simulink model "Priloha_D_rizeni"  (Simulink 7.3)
settings: Solver=ode45  StartTime=0.0  StopTime=0.7  FixedStep=0.6e-3  MaxStep=0.08e-3  RelTol=0.8e-3
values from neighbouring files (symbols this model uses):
  ILi = [0 Imax]    [Priloha_B_motor1_parametry.m]    (also in Priloha_C_motor2_parametry.m)
  Im = Psim / Ldi(1)    [Priloha_B_motor1_parametry.m]    (also in Priloha_C_motor2_parametry.m)
  Imax = 8    [Priloha_B_motor1_parametry.m]    (also in Priloha_C_motor2_parametry.m)
  J = 7e-3    (= 0.007)    [Priloha_B_motor1_parametry.m]    (also in Priloha_C_motor2_parametry.m)
  Kiid = 1 / (KM * 2 * tausigmaid / Rs)    (= 1975)    [Priloha_B_motor1_parametry.m]    (also in Priloha_C_motor2_parametry.m)
  Kiiq = 1 / (KM * 2 * tausigmaiq / Rs)    (= 1975)    [Priloha_B_motor1_parametry.m]    (also in Priloha_C_motor2_parametry.m)
  Kiwq = 1 / (Psim * p * 8 * (2 * tausigmaiq)^2 / J)    (= 306.115309264)    [Priloha_B_motor1_parametry.m]    (also in Priloha_C_motor2_parametry.m = 402.854511971)
  KM = 1    [Priloha_B_motor1_parametry.m]    (also in Priloha_C_motor2_parametry.m)
  Kpid = Ldi(1) / (KM * 2 * tausigmaid)    [Priloha_B_motor1_parametry.m]    (also in Priloha_C_motor2_parametry.m)
  Kpiq = Lqi(1) / (KM * 2 * tausigmaiq)    [Priloha_B_motor1_parametry.m]    (also in Priloha_C_motor2_parametry.m)
  Kpwq = 4 / (Psim * p * 8 * (2 * tausigmaiq) / J)    (= 2.44892247411)    [Priloha_B_motor1_parametry.m]    (also in Priloha_C_motor2_parametry.m = 3.22283609576)
  Ld = 22.5e-3    (= 0.0225)    [Priloha_B_motor1_parametry.m]    (also in Priloha_C_motor2_parametry.m)
  Ldi = [Ldi Ldi]    [Priloha_B_motor1_parametry.m]    (also in Priloha_C_motor2_parametry.m)
  Lq = 54e-3    (= 0.054)    [Priloha_B_motor1_parametry.m]    (also in Priloha_C_motor2_parametry.m)
  Lqi = [Lqi Lqi]    [Priloha_B_motor1_parametry.m]    (also in Priloha_C_motor2_parametry.m)
  p = 3    [Priloha_B_motor1_parametry.m]    (also in Priloha_C_motor2_parametry.m)
  Psim = 238.2e-3    (= 0.2382)    [Priloha_B_motor1_parametry.m]    (also in Priloha_C_motor2_parametry.m = 0.181)
  Rs = 3.95    [Priloha_B_motor1_parametry.m]    (also in Priloha_C_motor2_parametry.m)
  tausigmaid = 1 / fM    (= 0.001)    [Priloha_B_motor1_parametry.m]    (also in Priloha_C_motor2_parametry.m)
  tausigmaiq = 1 / fM    (= 0.001)    [Priloha_B_motor1_parametry.m]    (also in Priloha_C_motor2_parametry.m)
  Umax = 115    [Priloha_B_motor1_parametry.m]    (also in Priloha_C_motor2_parametry.m)
undefined symbols (not defined in the file or in its folder): Floor, magnitude
libraries: simulink x21
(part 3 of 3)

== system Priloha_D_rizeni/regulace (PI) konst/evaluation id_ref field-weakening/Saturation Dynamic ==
  up : Inport  OutDataType=fixdt(1, 16)  OutScaling=2^0
  u : Inport  Port=2  OutDataType=fixdt(1, 16)  OutScaling=2^0
  lo : Inport  Port=3  OutDataType=fixdt(1, 16)  OutScaling=2^0
  Data Type Duplicate : simulink/Signal Attributes/Data Type Duplicate  NumInputPorts=2
  Data Type Propagation : simulink/Signal Attributes/Data Type Propagation  PropDataType=fixdt(1, 16)  IfRefDouble=double  IfRefSingle=single  IsSigned=IsSigned1  NumBitsBase=NumBits1  NumBitsMult=1  NumBitsAdd=0  NumBitsAllowFinal=1:128  PropScaling=2^-10  ValuesUsedBestPrec=[5 -7]  SlopeBase=Slope1  SlopeMult=1  SlopeAdd=0  BiasBase=Bias1  BiasMult=1  BiasAdd=0
  LowerRelop1 : RelationalOperator  DisableCoverage=on  Operator=>  LogicOutDataTypeMode=boolean  LogicDataType=fixdt(0, 8)  OutDataTypeStr=boolean
  Switch : Switch  Criteria=u2 ~= 0  OutDataType=fixdt(1, 16)  OutScaling=2^0  OutDataTypeStr=Inherit: Inherit via back propagation  ZeroCross=off
  Switch2 : Switch  Criteria=u2 ~= 0  OutMin=OutMin  OutMax=OutMax  OutDataType=OutDataType  OutScaling=OutScaling  OutDataTypeStr=Inherit: Inherit via back propagation  ZeroCross=off
  UpperRelop : RelationalOperator  DisableCoverage=on  Operator=<  LogicOutDataTypeMode=boolean  LogicDataType=fixdt(0, 8)  OutDataTypeStr=boolean
  y1 : Outport  OutMin=OutMin  OutMax=OutMax  OutDataType=fixdt(1, 16)  OutScaling=2^0
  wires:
  up/1 -> Switch2/1, LowerRelop1/2
  u/1 -> Data Type Propagation/2, Data Type Propagation/1, LowerRelop1/1, Switch/3, UpperRelop/1
  lo/1 -> Switch/1, UpperRelop/2
  Switch/1 -> Data Type Duplicate/2, Switch2/3, Data Type Propagation/3
  Switch2/1 -> Data Type Duplicate/1, y1/1
  LowerRelop1/1 -> Switch2/2
  UpperRelop/1 -> Switch/2

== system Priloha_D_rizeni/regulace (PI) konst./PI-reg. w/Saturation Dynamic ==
  up : Inport  OutDataType=fixdt(1, 16)  OutScaling=2^0
  u : Inport  Port=2  OutDataType=fixdt(1, 16)  OutScaling=2^0
  lo : Inport  Port=3  OutDataType=fixdt(1, 16)  OutScaling=2^0
  Data Type Duplicate : simulink/Signal Attributes/Data Type Duplicate  NumInputPorts=2
  Data Type Propagation : simulink/Signal Attributes/Data Type Propagation  PropDataType=fixdt(1, 16)  IfRefDouble=double  IfRefSingle=single  IsSigned=IsSigned1  NumBitsBase=NumBits1  NumBitsMult=1  NumBitsAdd=0  NumBitsAllowFinal=1:128  PropScaling=2^-10  ValuesUsedBestPrec=[5 -7]  SlopeBase=Slope1  SlopeMult=1  SlopeAdd=0  BiasBase=Bias1  BiasMult=1  BiasAdd=0
  LowerRelop1 : RelationalOperator  DisableCoverage=on  Operator=>  LogicOutDataTypeMode=boolean  LogicDataType=fixdt(0, 8)  OutDataTypeStr=boolean
  Switch : Switch  Criteria=u2 ~= 0  OutDataType=fixdt(1, 16)  OutScaling=2^0  OutDataTypeStr=Inherit: Inherit via back propagation  ZeroCross=off
  Switch2 : Switch  Criteria=u2 ~= 0  OutMin=OutMin  OutMax=OutMax  OutDataType=OutDataType  OutScaling=OutScaling  OutDataTypeStr=Inherit: Inherit via back propagation  ZeroCross=off
  UpperRelop : RelationalOperator  DisableCoverage=on  Operator=<  LogicOutDataTypeMode=boolean  LogicDataType=fixdt(0, 8)  OutDataTypeStr=boolean
  y1 : Outport  OutMin=OutMin  OutMax=OutMax  OutDataType=fixdt(1, 16)  OutScaling=2^0
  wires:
  up/1 -> Switch2/1, LowerRelop1/2
  u/1 -> Data Type Propagation/2, Data Type Propagation/1, LowerRelop1/1, Switch/3, UpperRelop/1
  lo/1 -> Switch/1, UpperRelop/2
  Switch/1 -> Data Type Duplicate/2, Switch2/3, Data Type Propagation/3
  Switch2/1 -> Data Type Duplicate/1, y1/1
  LowerRelop1/1 -> Switch2/2
  UpperRelop/1 -> Switch/2

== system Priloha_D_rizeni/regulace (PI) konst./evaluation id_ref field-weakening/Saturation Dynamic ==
  up : Inport  OutDataType=fixdt(1, 16)  OutScaling=2^0
  u : Inport  Port=2  OutDataType=fixdt(1, 16)  OutScaling=2^0
  lo : Inport  Port=3  OutDataType=fixdt(1, 16)  OutScaling=2^0
  Data Type Duplicate : simulink/Signal Attributes/Data Type Duplicate  NumInputPorts=2
  Data Type Propagation : simulink/Signal Attributes/Data Type Propagation  PropDataType=fixdt(1, 16)  IfRefDouble=double  IfRefSingle=single  IsSigned=IsSigned1  NumBitsBase=NumBits1  NumBitsMult=1  NumBitsAdd=0  NumBitsAllowFinal=1:128  PropScaling=2^-10  ValuesUsedBestPrec=[5 -7]  SlopeBase=Slope1  SlopeMult=1  SlopeAdd=0  BiasBase=Bias1  BiasMult=1  BiasAdd=0
  LowerRelop1 : RelationalOperator  DisableCoverage=on  Operator=>  LogicOutDataTypeMode=boolean  LogicDataType=fixdt(0, 8)  OutDataTypeStr=boolean
  Switch : Switch  Criteria=u2 ~= 0  OutDataType=fixdt(1, 16)  OutScaling=2^0  OutDataTypeStr=Inherit: Inherit via back propagation  ZeroCross=off
  Switch2 : Switch  Criteria=u2 ~= 0  OutMin=OutMin  OutMax=OutMax  OutDataType=OutDataType  OutScaling=OutScaling  OutDataTypeStr=Inherit: Inherit via back propagation  ZeroCross=off
  UpperRelop : RelationalOperator  DisableCoverage=on  Operator=<  LogicOutDataTypeMode=boolean  LogicDataType=fixdt(0, 8)  OutDataTypeStr=boolean
  y1 : Outport  OutMin=OutMin  OutMax=OutMax  OutDataType=fixdt(1, 16)  OutScaling=2^0
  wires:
  up/1 -> Switch2/1, LowerRelop1/2
  u/1 -> Data Type Propagation/2, Data Type Propagation/1, LowerRelop1/1, Switch/3, UpperRelop/1
  lo/1 -> Switch/1, UpperRelop/2
  Switch/1 -> Data Type Duplicate/2, Switch2/3, Data Type Propagation/3
  Switch2/1 -> Data Type Duplicate/1, y1/1
  LowerRelop1/1 -> Switch2/2
  UpperRelop/1 -> Switch/2

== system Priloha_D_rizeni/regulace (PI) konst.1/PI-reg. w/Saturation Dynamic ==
  up : Inport  OutDataType=fixdt(1, 16)  OutScaling=2^0
  u : Inport  Port=2  OutDataType=fixdt(1, 16)  OutScaling=2^0
  lo : Inport  Port=3  OutDataType=fixdt(1, 16)  OutScaling=2^0
  Data Type Duplicate : simulink/Signal Attributes/Data Type Duplicate  NumInputPorts=2
  Data Type Propagation : simulink/Signal Attributes/Data Type Propagation  PropDataType=fixdt(1, 16)  IfRefDouble=double  IfRefSingle=single  IsSigned=IsSigned1  NumBitsBase=NumBits1  NumBitsMult=1  NumBitsAdd=0  NumBitsAllowFinal=1:128  PropScaling=2^-10  ValuesUsedBestPrec=[5 -7]  SlopeBase=Slope1  SlopeMult=1  SlopeAdd=0  BiasBase=Bias1  BiasMult=1  BiasAdd=0
  LowerRelop1 : RelationalOperator  DisableCoverage=on  Operator=>  LogicOutDataTypeMode=boolean  LogicDataType=fixdt(0, 8)  OutDataTypeStr=boolean
  Switch : Switch  Criteria=u2 ~= 0  OutDataType=fixdt(1, 16)  OutScaling=2^0  OutDataTypeStr=Inherit: Inherit via back propagation  ZeroCross=off
  Switch2 : Switch  Criteria=u2 ~= 0  OutMin=OutMin  OutMax=OutMax  OutDataType=OutDataType  OutScaling=OutScaling  OutDataTypeStr=Inherit: Inherit via back propagation  ZeroCross=off
  UpperRelop : RelationalOperator  DisableCoverage=on  Operator=<  LogicOutDataTypeMode=boolean  LogicDataType=fixdt(0, 8)  OutDataTypeStr=boolean
  y1 : Outport  OutMin=OutMin  OutMax=OutMax  OutDataType=fixdt(1, 16)  OutScaling=2^0
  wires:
  up/1 -> Switch2/1, LowerRelop1/2
  u/1 -> Data Type Propagation/2, Data Type Propagation/1, LowerRelop1/1, Switch/3, UpperRelop/1
  lo/1 -> Switch/1, UpperRelop/2
  Switch/1 -> Data Type Duplicate/2, Switch2/3, Data Type Propagation/3
  Switch2/1 -> Data Type Duplicate/1, y1/1
  LowerRelop1/1 -> Switch2/2
  UpperRelop/1 -> Switch/2

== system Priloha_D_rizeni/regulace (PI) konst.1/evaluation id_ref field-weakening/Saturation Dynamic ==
  up : Inport  OutDataType=fixdt(1, 16)  OutScaling=2^0
  u : Inport  Port=2  OutDataType=fixdt(1, 16)  OutScaling=2^0
  lo : Inport  Port=3  OutDataType=fixdt(1, 16)  OutScaling=2^0
  Data Type Duplicate : simulink/Signal Attributes/Data Type Duplicate  NumInputPorts=2
  Data Type Propagation : simulink/Signal Attributes/Data Type Propagation  PropDataType=fixdt(1, 16)  IfRefDouble=double  IfRefSingle=single  IsSigned=IsSigned1  NumBitsBase=NumBits1  NumBitsMult=1  NumBitsAdd=0  NumBitsAllowFinal=1:128  PropScaling=2^-10  ValuesUsedBestPrec=[5 -7]  SlopeBase=Slope1  SlopeMult=1  SlopeAdd=0  BiasBase=Bias1  BiasMult=1  BiasAdd=0
  LowerRelop1 : RelationalOperator  DisableCoverage=on  Operator=>  LogicOutDataTypeMode=boolean  LogicDataType=fixdt(0, 8)  OutDataTypeStr=boolean
  Switch : Switch  Criteria=u2 ~= 0  OutDataType=fixdt(1, 16)  OutScaling=2^0  OutDataTypeStr=Inherit: Inherit via back propagation  ZeroCross=off
  Switch2 : Switch  Criteria=u2 ~= 0  OutMin=OutMin  OutMax=OutMax  OutDataType=OutDataType  OutScaling=OutScaling  OutDataTypeStr=Inherit: Inherit via back propagation  ZeroCross=off
  UpperRelop : RelationalOperator  DisableCoverage=on  Operator=<  LogicOutDataTypeMode=boolean  LogicDataType=fixdt(0, 8)  OutDataTypeStr=boolean
  y1 : Outport  OutMin=OutMin  OutMax=OutMax  OutDataType=fixdt(1, 16)  OutScaling=2^0
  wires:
  up/1 -> Switch2/1, LowerRelop1/2
  u/1 -> Data Type Propagation/2, Data Type Propagation/1, LowerRelop1/1, Switch/3, UpperRelop/1
  lo/1 -> Switch/1, UpperRelop/2
  Switch/1 -> Data Type Duplicate/2, Switch2/3, Data Type Propagation/3
  Switch2/1 -> Data Type Duplicate/1, y1/1
  LowerRelop1/1 -> Switch2/2
  UpperRelop/1 -> Switch/2
